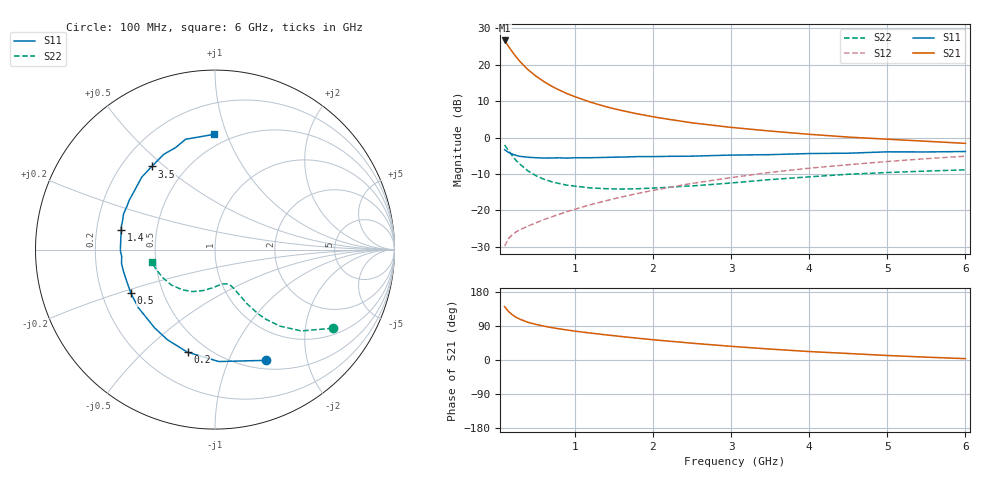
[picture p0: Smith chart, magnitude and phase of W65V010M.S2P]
! SIEMENS Small Signal Semiconductors
! BFR193W
! Si NPN RF Bipolar Junction Transistor in SOT323
! VCE = 5 V  IC = 10 mA
! Common Emitter S-Parameters:  September  1992
# GHz  S  MA  R  50
!  f  S11  S21  S12  S22
! GHz  MAG  ANG  MAG  ANG  MAG  ANG  MAG  ANG
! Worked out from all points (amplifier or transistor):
!   28 points, 100 MHz to 6 GHz, reference 50 ohm
!   highest |S21| = 26.7 dB at 100 MHz (marker M1)
!   |S21| within 3 dB of that: start of sweep to 194.7 MHz
!   unconditionally stable (mu >= 1): 1.017 GHz to 2.562 GHz
!   at 300 MHz: K = 0.55, MSG = 23.1 dB, |S12| = -25.3 dB
!   at 1.5 GHz: K = 1.05, MAG = 11.0 dB, |S12| = -16.9 dB
!   at 6 GHz: K = 0.89, MSG = 1.8 dB, |S12| = -5.1 dB
!   lowest NFmin = 1.30 dB at 450 MHz
!   S11 on the Smith chart (normalised r, x): 100 MHz: 0.60, -1.38; 200 MHz: 0.39, -0.69; 500 MHz: 0.33, -0.22; 1.4 GHz: 0.31, +0.09; 3.5 GHz: 0.32, +0.45; 6 GHz: 0.41, +0.90
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0.1  0.6797 -65.2  21.63 140.7  0.0321 61.7  0.7895 -33.7
0.15  0.6241 -88.0  17.94 128.0  0.0409 54.8  0.6607 -43.3
0.2  0.5918 -105.0  15.03 118.9  0.0464 51.2  0.5604 -49.6
0.25  0.568 -117.9  12.74 112.4  0.0507 49.2  0.4814 -53.8
0.3  0.5507 -127.7  11.02 107.2  0.0543 48.9  0.4269 -56.3
0.4  0.536 -142.8  8.582 99.5  0.0607 49.9  0.3477 -59.5
0.5  0.5282 -152.5  7.011 94.0  0.0671 51.7  0.2996 -61.1
0.6  0.5226 -160.1  5.916 89.5  0.0744 53.5  0.268 -62.7
0.7  0.524 -166.2  5.094 85.6  0.0809 55.6  0.2474 -63.6
0.8  0.5264 -171.6  4.498 82.2  0.0882 57.0  0.233 -65.0
0.9  0.5213 -175.8  4.012 79.1  0.0959 58.5  0.2215 -65.8
1  0.5275 -179.5  3.648 76.2  0.1034 59.7  0.2148 -67.3
1.2  0.5282 173.5  3.065 71.1  0.1193 61.4  0.2028 -70.6
1.4  0.5339 168.1  2.654 66.3  0.1355 62.4  0.1983 -74.1
1.8  0.5469 158.7  2.118 57.6  0.17 63.3  0.1978 -82.0
2.2  0.5517 149.8  1.782 49.8  0.2057 62.9  0.2071 -89.7
2.5  0.5552 144.4  1.594 44.3  0.2338 62.0  0.2161 -95.6
3  0.574 135.3  1.38 36.1  0.2816 59.6  0.2372 -106.0
3.5  0.582 127.2  1.228 28.8  0.332 56.4  0.2644 -117.8
4.5  0.6093 111.1  1.015 17.2  0.4231 48.3  0.3129 -140.8
5.5  0.6342 97.1  0.889 7.5  0.512 39.6  0.3461 -161.5
6  0.6426 90.4  0.832 3.6  0.5545 34.7  0.3595 -168.7
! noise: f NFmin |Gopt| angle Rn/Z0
0.45  1.3  0.22  143  0.11
0.9  1.3  0.34  160  0.11
1.8  2.05  0.54  -153  0.14
